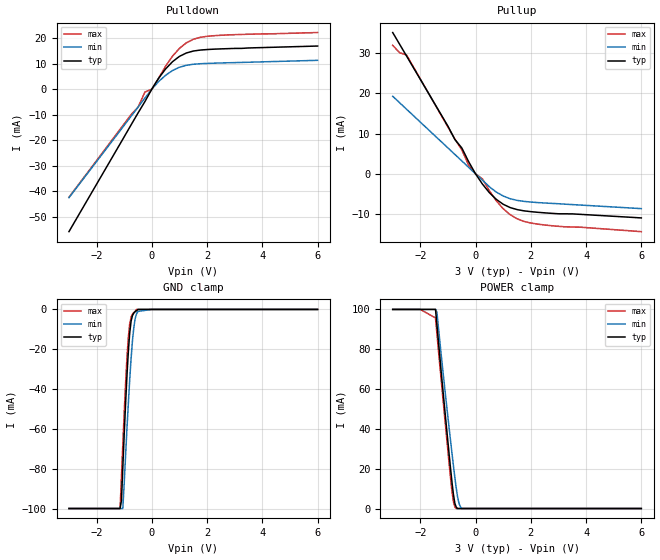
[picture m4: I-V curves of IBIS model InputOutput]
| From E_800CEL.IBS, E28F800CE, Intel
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|********************Input Output Model**************************
[Model]   InputOutput
Model_type   I/O
|   Model for DQ[0:15] pins.
Vinl = 0.8V
Vinh = 2.0V
|Variable   Typ   Min   Max
C_comp   9.61p   NA   11.6p
[Voltage Range]   3.0V   2.7V   3.3V
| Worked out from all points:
|   slope of the pulldown table from 0 to 0.45 V, typ, clamps not added: 62.4 ohm
|   slope of the pullup table from 0 to 0.45 V, typ, clamps not added: 106 ohm
|   GND clamp passes 1 mA (typ) near -0.59 V on its own axis
|   POWER clamp passes 1 mA (typ) near -0.71 V on its own axis
[Pulldown]
| [Pullup] and [Pulldown] IV curves include only the current through
| the channels of output driver transistors when outputs are enabled
| with OE# = VIL.  Although the output driver transistors have np and
| pn diodes inherently created by CMOS IC fabrication between the
| drain and bulk of n-channel and p-channel CMOS transistors,
| the current through these junction diodes is not included in
| [Pullup] or [Pulldown].  Instead that drain/bulk diode current is
| included in the [POWER_clamp] or [GND_clamp] sections, which are
| not dependent on the state of OE# or output data value.
|Voltage   I(typ)   I(min)   I(max)
-3V       -55.89mA   -42.58mA   -42.4mA
-750mV    -14mA      -10.63mA   -9.973mA
-500mV    -9.358mA   -7.089mA   -7.118mA
-250mV    -4.87mA    -3.473mA   -1.145mA
0V        0A         0A         0A
250mV     4.345mA    3.02mA     4.344mA
750mV     10.78mA    7.303mA    12.96mA
1V        12.85mA    8.592mA    16mA
1.25V     14.18mA    9.358mA    18.16mA
1.5V      14.94mA    9.758mA    19.54mA
2V        15.53mA    10.09mA    20.73mA
6V        16.9mA     11.3mA     22.2mA
[GND_clamp]
| [POWER_clamp] and [GND_clamp] IV curves describe ESD protection
| circuits PLUS some np and pn diodes which exist between the
| drain and bulk of n-channel and p-channel CMOS transistors.
| These drain/bulk diodes are inherent in CMOS IC fabrication,
| and are visible on the node of the I/O pin at all times.
| Even the drain/bulk diodes of output driver [Pullup] and [Powerdown]
| transistors are included in [POWER_clamp] or [GND_clamp], because
| these diodes contribute to I/O pin current even when the
| chip outputs are tristated by OE# = VIH.
| For example, when V forced on the I/O pin is large, we are
| forward biasing the pn diode at the drain/bulk interface in the
| p-channel pullup transistor.  Similarly, when V forced on the
| I/O pin is sufficiently negative with respect to the substrate
| ground, we are forward biasing the np diode at the drain/bulk
| interface in the n-channel pulldown transistor.  The effects
| of these diodes are included in [POWER_clamp] or [GND_clamp].
|Voltage   I(typ)   I(min)   I(max)
-3V       -100mA     -100mA     -100mA
-1.15V    -100mA     -100mA     -100mA
-1.1V     -96.13mA   -100mA     -84.28mA
-1.05V    -79.27mA   -100mA     -67.85mA
-900mV    -33.09mA   -59.72mA   -24.15mA
-850mV    -21.18mA   -47.23mA   -13.99mA
-800mV    -11.68mA   -35.18mA   -7.115mA
-750mV    -5.859mA   -24.53mA   -3.827mA
-650mV    -1.796mA   -8.797mA   -1.499mA
-550mV    -609.5uA   -2.086mA   0A
0V        0A         0A         0A
6V        0A         0A         0A
[Pullup]
| (Voltages for [Pullup] and [POWER_clamp] are specified with
| negative respect to Vcc.  Reference the IBIS documentation
| for more information regarding Vtable = Vcc - Voutput.
| This method keeps -Vds constant for the values in all three
| columns across a line of the table.
| [Pullup] and [Pulldown] IV curves include only the current through
| the channels of output driver transistors when outputs are enabled
| with OE# = VIL.  Although the output driver transistors have np and
| pn diodes inherently created by CMOS IC fabrication between the
| drain and bulk of n-channel and p-channel CMOS transistors,
| the current through these junction diodes is not included in
| [Pullup] or [Pulldown].  Instead that drain/bulk diode current is
| included in the [POWER_clamp] or [GND_clamp] sections, which are
| not dependent on the state of OE# or output data value.
|Voltage  I(typ)   I(min)   I(max)
-3V       35mA       19.22mA    31.83mA
-2.75V    32.1mA     17.62mA    30mA
-2.5V     29.2mA     16.02mA    29.45mA
-750mV    8.526mA    4.82mA     8.625mA
-500mV    6.438mA    3.22mA     5.968mA
-250mV    3.008mA    1.62mA     2.125mA
0V        0A         0A         0A
250mV     -2.54mA    -1.548mA   -1.258mA
750mV     -6.307mA   -4.501mA   -6.665mA
1.25V     -8.337mA   -6.145mA   -10.1mA
2V        -9.353mA   -6.97mA    -12.17mA
6V        -10.9mA    -8.6mA     -14.3mA
[POWER_clamp]
| (Voltages for [Pullup] and [POWER_clamp] are specified with
| negative respect to Vcc.  Reference the IBIS documentation
| for more information regarding Vtable = Vcc - Voutput.
| This method keeps -Vds constant for the values in all three
| columns across a line of the table.
| [POWER_clamp] and [GND_clamp] IV curves describe ESD protection
| circuits PLUS some np and pn diodes which exist between the
| drain and bulk of n-channel and p-channel CMOS transistors.
| These drain/bulk diodes are inherent in CMOS IC fabrication,
| and are visible on the node of the I/O pin at all times.
| Even the drain/bulk diodes of output driver [Pullup] and [Powerdown]
| transistors are included in [POWER_clamp] or [GND_clamp], because
| these diodes contribute to I/O pin current even when the
| chip outputs are tristated by OE# = VIH.
| For example, when V forced on the I/O pin is large, we are
| forward biasing the pn diode at the drain/bulk interface in the
| p-channel pullup transistor.  Similarly, when V forced on the
| I/O pin is sufficiently negative with respect to the substrate
| ground, we are forward biasing the np diode at the drain/bulk
| interface in the n-channel pulldown transistor.  The effects
| of these diodes are included in [POWER_clamp] or [GND_clamp].
|Voltage I(typ)   I(min)   I(max)
-3V       100mA      100mA      100mA
-2V       100mA      100mA      100mA
-1.45V    100mA      100mA      95.7mA
-1.4V     92.32mA    98.66mA    87.94mA
-1.15V    54.74mA    64.81mA    50.49mA
-900mV    19.28mA    33.34mA    14.38mA
-800mV    6.826mA    21.3mA     3.211mA
-750mV    2.604mA    15.54mA    747.1uA
-700mV    636.3uA    10.25mA    0A
-600mV    0A         2.578mA    0A
-500mV    0A         0A         0A
6V        0A         0A         0A
[Ramp]
| The DQ Ramp information is not provided at this time for the
| device but will be available in the future.  The table below
| is for the compatibility with some IBIS parsers.
| Variable   typ   min   max
 dV/dt_r   0V/0ns   0V/0ns   0V/0ns
 dV/dt_f   0V/0ns   0V/0ns   0V/0ns
